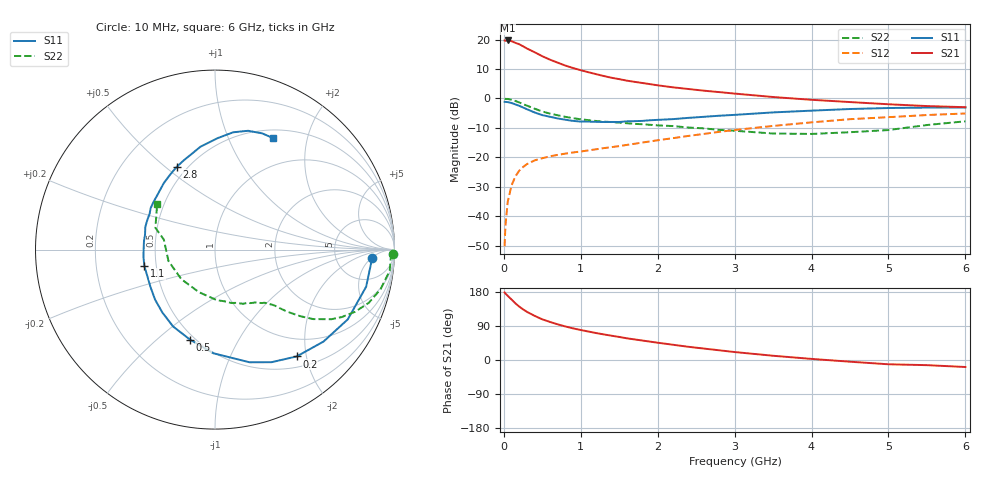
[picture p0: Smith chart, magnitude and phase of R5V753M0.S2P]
! SIEMENS Small Signal Semiconductors
! BFR183
! Si NPN RF Bipolar Junction Transistor in SOT23
! VCE = 0.75 V  IC = 3 mA
! Common Emitter S-Parameters:  May  1996
# GHz  S  MA  R  50
!  f  S11  S21  S12  S22
! GHz  MAG  ANG  MAG  ANG  MAG  ANG  MAG  ANG
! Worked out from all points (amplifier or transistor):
!   36 points, 10 MHz to 6 GHz, reference 50 ohm
!   highest |S21| = 19.7 dB at 50 MHz (marker M1)
!   |S21| within 3 dB of that: start of sweep to 321.5 MHz
!   unconditionally stable (mu >= 1): 1.182 GHz to 3.14 GHz
!   at 250 MHz: K = 0.31, MSG = 20.5 dB, |S12| = -23.3 dB
!   at 1.4 GHz: K = 1.07, MAG = 10.1 dB, |S12| = -16.5 dB
!   at 6 GHz: K = 0.96, MSG = 1.1 dB, |S12| = -5.1 dB
!   S11 on the Smith chart (normalised r, x): 10 MHz: 13, -5; 200 MHz: 0.67, -1.83; 500 MHz: 0.47, -0.65; 1.1 GHz: 0.43, -0.09; 2.8 GHz: 0.44, +0.55; 6 GHz: 0.60, +1.48
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0.01  0.8745 -2.9  9.627 178.2  0.0031 89.4  0.9917 -1.4
0.02  0.8723 -5.4  9.545 175.7  0.0067 87.4  0.9804 -2.7
0.05  0.8671 -13.8  9.65 169.6  0.0175 83.1  0.9805 -6.9
0.1  0.8358 -27.7  9.381 159.6  0.0333 75.2  0.949 -13.4
0.15  0.7924 -40.3  8.791 149.5  0.0474 68.3  0.9065 -19.1
0.2  0.7492 -52.6  8.326 141.0  0.0593 63.1  0.8541 -23.9
0.25  0.7021 -63.3  7.677 133.6  0.0685 58.3  0.8005 -28.0
0.3  0.6565 -73.0  7.051 127.1  0.0767 55.1  0.7553 -30.9
0.4  0.5777 -90.9  6.087 116.5  0.0887 49.9  0.67 -35.3
0.5  0.5207 -105.4  5.213 107.3  0.0966 46.8  0.5998 -38.1
0.6  0.4881 -118.5  4.555 100.4  0.1041 44.8  0.5526 -39.8
0.7  0.4573 -129.8  4.05 94.1  0.11 43.8  0.5177 -41.1
0.8  0.435 -140.1  3.614 88.5  0.1156 43.4  0.4868 -42.1
1.1  0.4042 -166.9  2.785 75.1  0.1312 44.8  0.4279 -45.1
1.3  0.3977 179.8  2.401 67.5  0.1433 45.6  0.4039 -47.1
1.6  0.4084 161.9  2.003 57.2  0.1626 46.8  0.3794 -51.4
2.2  0.4455 135.1  1.543 40.2  0.2117 47.7  0.3394 -62.8
2.8  0.5085 114.7  1.281 25.6  0.2709 44.9  0.2921 -80.0
3.5  0.5791 98.0  1.057 11.2  0.3413 38.1  0.2536 -110.6
4.5  0.6614 81.2  0.868 -4.5  0.4443 25.6  0.267 -166.3
5.5  0.6989 67.9  0.742 -13.6  0.5226 13.0  0.3536 159.9
6  0.7006 62.4  0.71 -18.5  0.5554 4.8  0.4091 142.0
